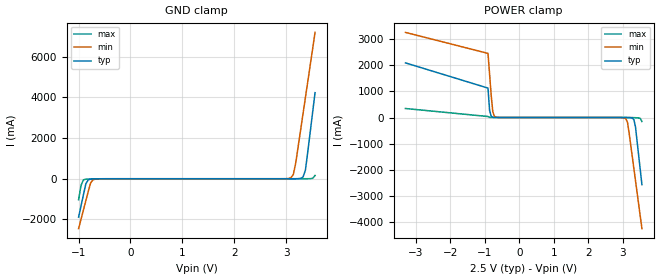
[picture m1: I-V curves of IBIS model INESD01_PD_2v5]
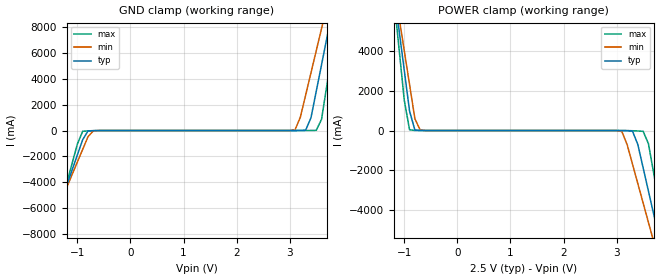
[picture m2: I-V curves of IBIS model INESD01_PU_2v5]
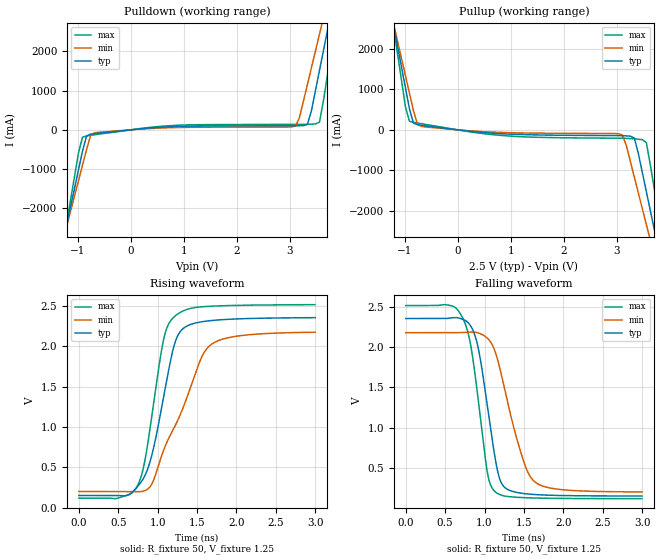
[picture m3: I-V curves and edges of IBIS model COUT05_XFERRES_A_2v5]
|   This file is an IBIS representation of the   |
|   Integrated Device Technology, Inc.   |
|   ICS83021I   |
|   1-TO-1 DIFFERENTIAL- TO-LVCMOS/LVTTL TRANSLATOR   |
[IBIS Ver]   4.1
[File name]   83021i.ibs
[File Rev]   1.0
[Date]   23 Nov 2009 | Last modified
|   Sep 11 2006 | Generated
[Source]   Originated at Integrated Device Technology, Inc.
[Disclaimer]
IDT hereby grants the user of this IBIS model a non-exclusive,
nontransferable license to use this IBIS model under the following terms.
Before using this IBIS model, the user should read this license.
If the user does not accept these terms,  the IBIS model should be
returned to IDT within 30 days.
   The user is granted this license only to use the IBIS model and
is not granted rights to sell, load, rent, lease or license the IBIS
model in whole or in part, or in modified form to anyone other than
user. User may modify the IBIS model to suit its specific
applications but rights to derivative works and such modifications
shall belong to IDT.
   This IBIS model is provided on an "AS IS" basis and IDT makes
absolutely no warranty with respect to the information contained
herein. IDT DISCLAIMS AND CUSTOMER WAIVES ALL WARRANTIES, EXPRESS
OR IMPLIED, INCLUDING WARRANTIES OF MERCHANTABILITY OR FITNESS FOR
A PARTICULAR PURPOSE. The entire risk as to quality and performance
is with the Customer. ACCORDINGLY, IN NO EVENT SHALL THE COMPANY BE
LIABLE FOR ANY DAMAGES, WHETHER IN CONTRACT OR TORT,INCLUDING ANY
LOST PROFITS OR OTHER INCIDENTAL, CONSEQUENTIAL, EXEMPLARY, OR
PUNITIVE DAMAGES ARISING OUT OF THE USE OR APPLICATION OF THE IBIS
model provided in this package. Further, IDT reserves the right to
make changes without notice to any product herein to improve
reliability, function, or design. IDT does not convey any license
under patent rights or any other intellectual property rights,
including those of third parties.
   IDT is not obligated to provide maintenance or support
for the licensed IBIS model.
[Copyright]   Copyright 2006 by Integrated Device Technology, Inc.
[Component]   ICS83021AMI
[Manufacturer] Integrated Device Technology, Inc.
[Package]
|SOIC 8 Lead
|   typ   min   max
R_pkg   57.05m   55.5m   58.6m
L_pkg   1.769nH   1.570nH   1.968nH
C_pkg   0.269pF   0.252pF   0.286pF
[Pin] signal_name  model_name   R_pin   L_pin   C_pin
1   NC   NC   58.6m   1.968n   0.286p
2   CLK   INESD01_PD   55.5m   1.570n   0.252p
3   nCLK   INESD01_PU   55.5m   1.570n   0.252p
4   NC   NC   56.6m   1.968n   0.286p
5   GND   GND   58.6m   1.968n   0.286p
6   NC   NC   55.5m   1.570n   0.252p
7   Q0   COUT05_XFERRES_A   55.5m   1.570n   0.252p
8   VDD   POWER   56.6m   1.968n   0.286p
[Diff Pin]  inv_pin  vdiff tdelay_typ tdelay_min  tdelay_max
2   3   NA   0  0  0
[Model Selector] INESD01_PD
INESD01_PD_2v5  Buffer selection for 2v5
INESD01_PD_3v3  Buffer selection for 3v3
[Model Selector] INESD01_PU
INESD01_PU_2v5  Buffer selection for 2v5
INESD01_PU_3v3  Buffer selection for 3v3
[Model Selector] COUT05_XFERRES_A
COUT05_XFERRES_A_2v5  Buffer selection for 2v5
COUT05_XFERRES_A_3v3  Buffer selection for 3v3
| Models and submodels in the file (6): INESD01_PD_2v5 (Input), INESD01_PU_2v5 (Input), COUT05_XFERRES_A_2v5 (Output), INESD01_PD_3v3 (Input), INESD01_PU_3v3 (Input), COUT05_XFERRES_A_3v3 (Output)
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[Model] INESD01_PD_2v5
Model_type   Input
Polarity   Non-Inverting
Vinl = 0.8V
Vinh = 2.0V
|   typ   min   max
C_comp   2pF   1.5pF   2.5pF
|   typ   min   max
[Voltage range]  2.5V   2.375V   2.625V
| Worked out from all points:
|   GND clamp passes 1 mA (typ) near -0.55 V on its own axis
|   POWER clamp passes 1 mA (typ) near -0.68 V on its own axis
[GND_clamp]
|Voltage I(typ)   I(min)   I(max)
-1V       -1.886A    -2.451A    -1.028A
-953.5mV  -1.338A    -1.994A    -328mA
-907mV    -789.6mA   -1.537A    -53.04mA
-860.5mV  -251.4mA   -1.081A    -21.51mA
-767.5mV  -17.28mA   -198.8mA   -10.01mA
-674.5mV  -5.28mA    -15.38mA   -3.684mA
3.092V    224.5uA    49.06mA    51.52uA
3.139V    500.8uA    208.3mA    52.98uA
3.185V    1.252mA    774.6mA    56.66uA
3.325V    81.55mA    3.177A     200uA
3.371V    416.9mA    3.978A     464.6uA
3.557V    4.225A     7.185A     159.2mA
[POWER_clamp]
|Voltage   I(typ)   I(min)   I(max)
-3.3V     2.083A     3.246A     343.1mA
-907mV    1.122A     2.445A     37.78mA
-860.5mV  267.5mA    1.644A     5.973mA
-814mV    47.03mA    844mA      1.727mA
-767.5mV  9.66mA     215.3mA    677uA
-674.5mV  960.6uA    12.66mA    131.4uA
3.092V    -1.849mA   -49.09mA   -51.51uA
3.139V    -3.491mA   -186mA     -159.7uA
3.325V    -84.03mA   -1.955A    -5.102mA
3.371V    -365.4mA   -2.411A    -8.31mA
3.51V     -2.01A     -3.782A    -35.44mA
3.557V    -2.558A    -4.239A    -152.3mA
[Model] INESD01_PU_2v5
Model_type   Input
Polarity   Non-Inverting
Vinl = 1.4V
Vinh = 1.85V
|   typ   min   max
C_comp   2pF   1.5pF   2.5pF
|   typ   min   max
[Voltage range]  2.5V   2.375V   2.625V
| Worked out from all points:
|   GND clamp passes 1 mA (typ) near -0.54 V on its own axis
|   POWER clamp passes 1 mA (typ) near -0.66 V on its own axis
[GND_clamp]
|Voltage   I(typ)   I(min)   I(max)
-2.5V     -19.6A     -17.18A    -23.67A
-1.6V     -8.969A    -8.332A    -10.1A
-1.5V     -7.788A    -7.349A    -8.588A
-900mV    -707.1mA   -1.46A     -57.43mA
-700mV    -7.027mA   -24.05mA   -13.28mA
3.1V      199.2uA    53.94mA    11.78uA
3.3V      28.4mA     2.748A     652.4uA
3.5V      3.045A     6.192A     15.72mA
3.6V      5.115A     7.914A     872.4mA
3.7V      7.185A     9.638A     3.52A
3.9V      11.33A     13.09A     8.818A
5V        34.14A     32.07A     37.99A
[POWER_clamp]
|Voltage   I(typ)   I(min)   I(max)
-1.5V     9.257A     9.207A     9.48A
-1.2V     7.185A     7.484A     6.83A
-1.1V     5.115A     5.761A     4.182A
-900mV    976.9mA    2.318A     34.23mA
-700mV    1.582mA    24.31mA    1.044mA
3.1V      -2.107mA   -51.03mA   -534.5uA
3.3V      -35.62mA   -1.705A    -10.86mA
3.5V      -1.886A    -3.666A    -39.41mA
3.6V      -3.066A    -4.647A    -666.9mA
3.8V      -5.426A    -6.612A    -3.684A
3.9V      -6.607A    -7.595A    -5.193A
5V        -19.6A     -18.41A    -21.79A
[Model] COUT05_XFERRES_A_2v5
Model_type  Output
Polarity   Non-Inverting
Vmeas = 1.25
Rref = 50
Cref = 0
Vref = 1.25
|Variable  typ   min   max
C_comp   2p   1.5p   2.5p
[Voltage Range]   2.5   2.375   2.625
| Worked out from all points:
|   slope of the pulldown table from 0 to 0.375 V, typ, clamps not added: 7.84 ohm
|   slope of the pullup table from 0 to 0.375 V, typ, clamps not added: 7.17 ohm
|   rising waveform, R_fixture 50, V_fixture 1.25: 20-80 % time 274ps typ, 488ps min, 225ps max; typ from 0.154 V to 2.35 V
|   falling waveform, R_fixture 50, V_fixture 1.25: 20-80 % time 205ps typ, 309ps min, 191ps max; typ from 2.35 V to 0.154 V
| Open source, no load
|  Voltage   I(typ)   I(min)   I(max)
[Pullup]
-2.5V     11.44A     9.986A     13.84A
-1.212V   2.607A     2.64A      2.573A
-909.1mV  526mA      911.1mA    212mA
-833.3mV  167.1mA    478.9mA    184.4mA
-681.8mV  112.7mA    84.76mA    151.8mA
3.106V    -144.5mA   -124.8mA   -207.2mA
3.333V    -201.9mA   -1.16A     -222.3mA
3.485V    -1.051A    -1.943A    -242.2mA
3.561V    -1.521A    -2.334A    -315mA
3.712V    -2.464A    -3.118A    -1.472A
3.864V    -3.407A    -3.903A    -2.677A
5V        -10.49A    -9.798A    -11.71A
[Pulldown]
-2.5V     -10.49A    -9.183A    -12.66A
-1.288V   -2.917A    -2.872A    -3.01A
-1.212V   -2.443A    -2.477A    -2.405A
-909.1mV  -543.8mA   -898.7mA   -186.9mA
-833.3mV  -160.7mA   -504.4mA   -155.1mA
-757.6mV  -109mA     -149.4mA   -139.6mA
3.106V    103.9mA    93.06mA    139.6mA
3.333V    137.9mA    1.155A     141.5mA
3.561V    1.512A     2.434A     197.9mA
3.712V    2.539A     3.288A     1.405A
3.864V    3.567A     4.143A     2.72A
5V        11.31A     10.58A     12.63A
[Ramp]
|   typ   min   max
dV/dt_r   1.762/0.433n   1.577/0.660n   1.919/0.360n
dV/dt_f   1.769/0.311n   1.585/0.457n   1.923/0.297n
R_load =   50.0000
[Rising Waveform]
R_fixture = 50
V_fixture = 1.25   | VCC_typ
V_fixture_max = 1.3125   | VCC_max
V_fixture_min = 1.1875   | VCC_min
C_fixture = 0.0p
| Time   typ   min   max
0s        154.1mV    203.2mV    121.3mV
477.4ps   154.3mV    203.2mV    116.6mV
740.9ps   259.7mV    200.8mV    269.6mV
821.5ps   368.8mV    208.9mV    507.2mV
905.2ps   578.3mV    264.4mV    996.6mV
1.079ns   1.39V      722.9mV    2.098V
1.228ns   2.067V     1.027V     2.379V
1.553ns   2.301V     1.854V     2.487V
1.693ns   2.318V     2.03V      2.495V
2.998ns   2.352V     2.173V     2.513V
[Falling Waveform]
R_fixture = 50
V_fixture = 1.25   | VCC_typ
V_fixture_max = 1.3125   | VCC_max
V_fixture_min = 1.1875   | VCC_min
C_fixture = 0.0p
| Time   typ   min   max
0s        2.355V     2.179V     2.515V
725.4ps   2.344V     2.181V     2.356V
818.4ps   2.271V     2.187V     2.053V
911.4ps   2.026V     2.178V     1.415V
1.039ns   1.249V     2.109V     432mV
1.141ns   587mV      1.926V     202.8mV
1.259ns   258.4mV    1.464V     154.1mV
1.479ns   187.7mV    638mV      135.2mV
1.624ns   173.7mV    341.8mV    130.1mV
2.998ns   154.5mV    205mV      121.5mV
